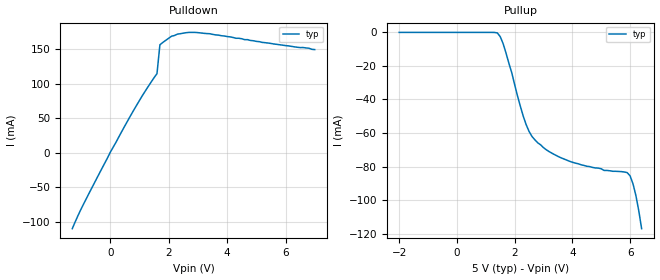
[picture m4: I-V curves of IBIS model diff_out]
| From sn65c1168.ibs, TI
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|   diff_out Model
[Model]   diff_out
Model_type   Output
Polarity   Non-Inverting
Vmeas = 2.05
Vref = 2.05
Cref = 2pF
Rref = 50
|   typ   min   max
C_comp   15pF   NA   NA
| Where Nom  PVT is Nominal Process, 5V, 27C
[Voltage Range]   5   NA   NA
|Junction Temperature
[Temperature Range]   27   NA   NA
[Pullup Reference]   5   NA   NA
[Pulldown Reference]   0   NA   NA
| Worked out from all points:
|   slope of the pulldown table from 0 to 0.75 V, typ, clamps not added: 13.1 ohm
[Pulldown]
|   Voltage   I(typ)   I(min)   I(max)
-1.3V     -109.8mA   NA         NA
-1V       -81.5mA    NA         NA
0V        800uA      NA         NA
900mV     68.8mA     NA         NA
1.6V      114.8mA    NA         NA
1.7V      156.6mA    NA         NA
1.8V      160mA      NA         NA
2.1V      169mA      NA         NA
2.3V      172mA      NA         NA
2.9V      174.5mA    NA         NA
3.4V      172.6mA    NA         NA
7V        149.6mA    NA         NA
[Pullup]
|  Voltage   I(typ)   I(min)   I(max)
-2V       0A         NA         NA
1.4V      -300uA     NA         NA
1.6V      -6.6mA     NA         NA
2.3V      -50mA      NA         NA
2.6V      -62mA      NA         NA
3.1V      -70mA      NA         NA
3.9V      -76.8mA    NA         NA
5.1V      -82.3mA    NA         NA
5.9V      -83.6mA    NA         NA
6.1V      -90.2mA    NA         NA
6.2V      -97.1mA    NA         NA
6.4V      -117mA     NA         NA
[Ramp]
R_load = 50
|   typ   min   max
dV/dt_r   2.044/0.92e-09   NA   NA
dV/dt_f   2.048/2.43e-09   NA   NA
